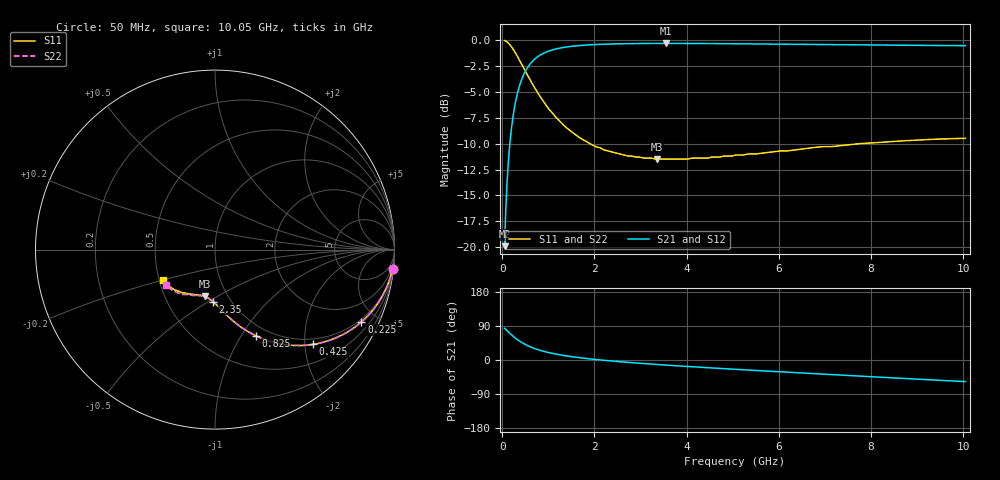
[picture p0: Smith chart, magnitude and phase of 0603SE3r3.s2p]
! AVX Thin Film Operation		Date: August 2001
! Description: Accu-P® Series, Thin Film, SMD, RF Capacitor
! Part Number: 06035J3R3ABT
! 50 MHz  -  10.05 GHz
! Serial Measurements
# mhz S db R 50
!	S11		S21		S12		S22
!	dB	Phase	dB	Phase	dB	Phase	dB	Phase
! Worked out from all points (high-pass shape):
!   401 points, 50 MHz to 10.05 GHz, reference 50 ohm
!   highest |S21| = -0.33 dB at 3.55 GHz (marker M1); lowest = -19.9 dB at 50 MHz (marker M2)
!   |S21| within 3 dB of the highest: 465 MHz to end of sweep
!   lowest |S11| = -11.5 dB at 3.35 GHz (marker M3), VSWR 1.73, Z = 39.3 - j22 ohm
!   |S11| at or under -10 dB: 1.902 GHz to 7.764 GHz (5.862 GHz wide, 121 % of centre)
!   |S22| runs from -11.5 to 0.0 dB; largest |S21 - S12| = 0
!   S11 on the Smith chart (normalised r, x): 50 MHz: 1, -18; 225 MHz: 0.88, -4.10; 425 MHz: 0.87, -2.18; 825 MHz: 0.87, -1.16; 2.35 GHz: 0.83, -0.52; 10.05 GHz: 0.52, -0.20
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50  -0.04 -6.2  -19.90 83.8  -19.90 83.8  -0.04 -6.2
75  -0.10 -9.3  -16.41 80.7  -16.41 80.7  -0.10 -9.3
125  -0.27 -15.3  -12.16 74.6  -12.16 74.6  -0.27 -15.3
150  -0.39 -18.3  -10.68 71.7  -10.68 71.7  -0.39 -18.3
175  -0.52 -21.0  -9.51 69.0  -9.51 69.0  -0.52 -21.0
225  -0.82 -26.3  -7.65 63.6  -7.65 63.6  -0.82 -26.4
325  -1.56 -35.9  -5.21 54.0  -5.21 54.0  -1.56 -35.9
425  -2.38 -44.0  -3.75 46.0  -3.75 46.0  -2.38 -44.0
525  -3.21 -50.6  -2.82 39.3  -2.82 39.3  -3.21 -50.6
625  -4.03 -56.1  -2.19 33.9  -2.19 33.9  -4.03 -56.1
825  -5.49 -64.7  -1.45 25.3  -1.45 25.3  -5.49 -64.6
1000  -6.61 -70.4  -1.07 19.6  -1.07 19.6  -6.61 -70.3
1200  -7.63 -75.2  -0.83 14.7  -0.83 14.7  -7.62 -75.1
1725  -9.55 -84.7  -0.52 5.3  -0.52 5.3  -9.55 -84.5
2350  -10.77 -92.5  -0.39 -2.4  -0.39 -2.4  -10.77 -92.0
3350  -11.50 -102.2  -0.33 -11.8  -0.33 -11.8  -11.42 -101.2
3400  -11.50 -102.8  -0.33 -12.2  -0.33 -12.2  -11.48 -101.8
3550  -11.50 -103.6  -0.33 -13.5  -0.33 -13.5  -11.50 -102.6
5050  -11.12 -115.8  -0.36 -24.6  -0.36 -24.6  -11.12 -113.0
6725  -10.40 -127.0  -0.43 -35.8  -0.43 -35.8  -10.40 -124.0
8400  -9.81 -139.1  -0.50 -46.6  -0.50 -46.6  -9.78 -134.1
10050  -9.49 -149.6  -0.55 -56.9  -0.55 -56.9  -9.45 -143.8
